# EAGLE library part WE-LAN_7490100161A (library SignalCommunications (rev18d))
WE-LAN LAN Transformer 10/100 Base T - Compliant with IEEE 802.3, IEEE 802.3af and IEEE 802.3at standards - SMT -- Ethernet -- Power over Ethernet -- 1 Gigabit Ethernet -- Compliant with most IC's for ethernet applications like Intel, AMD, Globespan and Realtek -- Hub, Router, Switch Details see: http://katalog.we-online.de/en/pbs/WE-LAN/7490100161A 2016 (C) Würth Elektronik
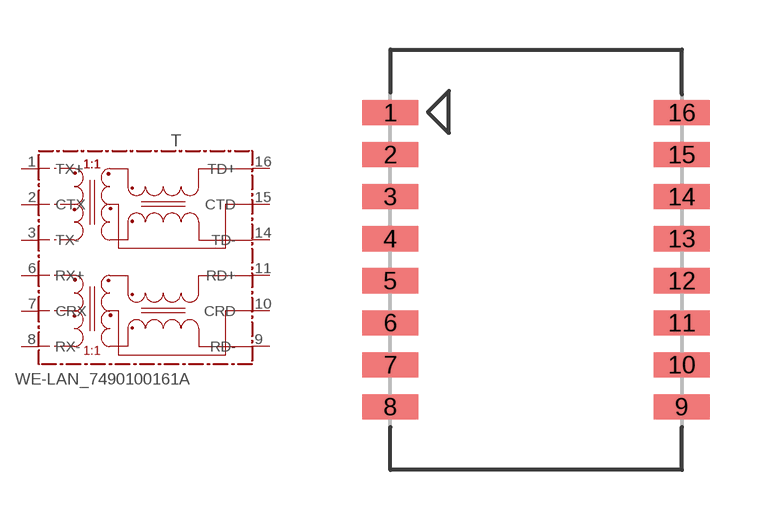
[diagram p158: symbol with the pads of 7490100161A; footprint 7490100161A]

Designator prefix T

## WE-LAN_7490100161A  [7490100161A]
1  TX+
2  CTX
3  TX-
6  RX+
7  CRX
8  RX-
9  RD-
10  CRD
11  RD+
14  TD-
15  CTD
16  TD+

## Footprint 7490100161A (pad centres in mm)
smd 1.7 x 0.76: 1 -4.4,4.445; 2 -4.4,3.175; 3 -4.4,1.905; 4 -4.4,0.635; 5 -4.4,-0.635; 6 -4.4,-1.905; 7 -4.4,-3.175; 8 -4.4,-4.445; 9 4.4,-4.445; 10 4.4,-3.175; 11 4.4,-1.905; 12 4.4,-0.635; 13 4.4,0.635; 14 4.4,1.905; 15 4.4,3.175; 16 4.4,4.445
